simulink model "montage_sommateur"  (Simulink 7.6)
settings: Solver=ode15s  StartTime=0.0  StopTime=0.2  RelTol=1e-3
InitFcn:
  | Ad=10^5;
  | Vsat=15;
StopFcn:
  | close all, clc
  | load  ES_sommateur.mat
  | plot(x(1,:),x(2,:))
  | hold on
  | plot(x(1,:),x(3,:))
  | plot(x(1,:),x(4,:))
  | grid
  | title('Tensions d'entrée et de sortie - Montage sommateur')
  | xlabel('temps')
libraries: fl_lib x23, nesl_utility x4

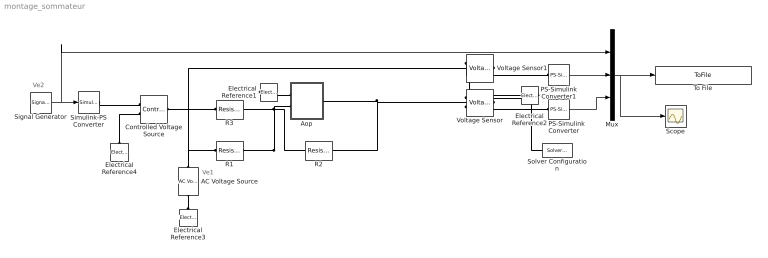
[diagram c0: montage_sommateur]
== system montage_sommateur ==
  note: Ve1
  note: Ve2
  AC Voltage Source : fl_lib/Electrical/Electrical Sources/AC Voltage Source  DialogController=NetworkEngine.DynNeDlgSource  SystemSampleTime=-1  amp=2 V  shift=0 rad  omega=10 Hz  i_Log=off  v_Log=off  LocalVarNames=|current|voltage|power  LocalVarDescs=|Current (A)|Voltage (V)|Power (W)  LocalVarLogging=[0 0 0]
  Aop : Subsystem
  Controlled Voltage Source : fl_lib/Electrical/Electrical Sources/Controlled Voltage Source  DialogController=NetworkEngine.DynNeDlgSource  SystemSampleTime=-1  i_Log=off  v_Log=off  LocalVarNames=|i|v  LocalVarDescs=|i|v  LocalVarLogging=[0 0]
  Electrical Reference{1..4} (4 alike) : fl_lib/Electrical/Electrical Elements/Electrical Reference  DialogController=NetworkEngine.DynNeDlgSource  SystemSampleTime=-1  i_Log=off  LocalVarNames=|i  LocalVarDescs=|i  LocalVarLogging=[]
  Mux : Mux  Inputs=3
  PS-Simulink Converter : nesl_utility/PS-Simulink Converter  DialogController=NetworkEngine.DynNeUtilDlgSource  SystemSampleTime=-1  PhysicalDomain=network_engine_domain  LeftPortType=input  RightPortType=output  SubClassName=ps_output  Unit=1  AffineConversion=off
  PS-Simulink Converter1 : nesl_utility/PS-Simulink Converter  DialogController=NetworkEngine.DynNeUtilDlgSource  SystemSampleTime=-1  PhysicalDomain=network_engine_domain  LeftPortType=input  RightPortType=output  SubClassName=ps_output  Unit=1  AffineConversion=off
  R1 : fl_lib/Electrical/Electrical Elements/Resistor  DialogController=NetworkEngine.DynNeDlgSource  SystemSampleTime=-1  R=10 kOhm  i_Log=off  v_Log=off  LocalVarNames=|current|voltage|power  LocalVarDescs=|Resistor current (A)|Voltage across resistor (V)|Power (W)  LocalVarLogging=[0 0 0]
  R2 : fl_lib/Electrical/Electrical Elements/Resistor  DialogController=NetworkEngine.DynNeDlgSource  SystemSampleTime=-1  R=10 kOhm  i_Log=off  v_Log=off  LocalVarNames=|current|voltage|power  LocalVarDescs=|Resistor current (A)|Voltage across resistor (V)|Power (W)  LocalVarLogging=[0 0 0]
  R3 : fl_lib/Electrical/Electrical Elements/Resistor  DialogController=NetworkEngine.DynNeDlgSource  SystemSampleTime=-1  R=10 kOhm  i_Log=off  v_Log=off  LocalVarNames=|current|voltage|power  LocalVarDescs=|Resistor current (A)|Voltage across resistor (V)|Power (W)  LocalVarLogging=[0 0 0]
  Scope : Scope
  Signal Generator : SignalGenerator  Frequency=20
  Simulink-PS Converter : nesl_utility/Simulink-PS Converter  DialogController=NetworkEngine.DynNeUtilDlgSource  SystemSampleTime=-1  PhysicalDomain=network_engine_domain  LeftPortType=input  RightPortType=output  SubClassName=ps_input  Unit=1  AffineConversion=off  InputFilterTimeConstant=.001  UdotUserProvided=0
  Solver Configuration : nesl_utility/Solver Configuration  DialogController=NetworkEngine.DynNeUtilDlgSource  SystemSampleTime=-1  PhysicalDomain=network_engine_domain  LeftPortType=input  RightPortType=generic  SubClassName=solver  Accelerate=off  Profile=off  ResidualTolerance=1e-9  MaxNonlinIter=12  MaxModeIter=2  DoFixedCost=off  UseLocalSampling=off  DoDC=off  LinearAlgebra=Sparse  LocalSolverSampleTime=.001  LocalSolverChoice=NE_BACKWARD_EULER_ADVANCER  UseLocalSolver=off
  To File : ToFile  Filename=ES_sommateur  MatrixName=x
  Voltage Sensor : fl_lib/Electrical/Electrical Sensors/Voltage Sensor  DialogController=NetworkEngine.DynNeDlgSource  SystemSampleTime=-1  i1_Log=off  v1_Log=off  LocalVarNames=|i1|v1  LocalVarDescs=|i1|v1  LocalVarLogging=[0 0]
  Voltage Sensor1 : fl_lib/Electrical/Electrical Sensors/Voltage Sensor  DialogController=NetworkEngine.DynNeDlgSource  SystemSampleTime=-1  i1_Log=off  v1_Log=off  LocalVarNames=|i1|v1  LocalVarDescs=|i1|v1  LocalVarLogging=[0 0]
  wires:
  Mux/1 -> To File/1, Scope/1
  Signal Generator/1 -> Simulink-PS Converter/1, Mux/1
  PS-Simulink Converter/1 -> Mux/3
  PS-Simulink Converter1/1 -> Mux/2
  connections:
  AC Voltage Source/RConn1 -- Electrical Reference3/LConn1
  Aop/RConn1 -- Voltage Sensor/LConn1 -- R2/RConn1
  Voltage Sensor/RConn1 -- PS-Simulink Converter/LConn1 -- Solver Configuration/RConn1
  Voltage Sensor/RConn2 -- Electrical Reference2/LConn1 -- Voltage Sensor1/RConn2
  R2/LConn1 -- R1/RConn1 -- Aop/LConn2 -- R3/RConn1
  Voltage Sensor1/RConn1 -- PS-Simulink Converter1/LConn1
  AC Voltage Source/LConn1 -- R1/LConn1 -- Voltage Sensor1/LConn1
  Electrical Reference1/LConn1 -- Aop/LConn1
  Controlled Voltage Source/LConn1 -- R3/LConn1
  Simulink-PS Converter/RConn1 -- Controlled Voltage Source/RConn1
  Electrical Reference4/LConn1 -- Controlled Voltage Source/RConn2

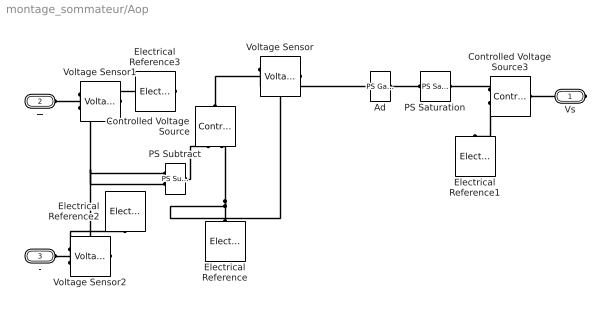
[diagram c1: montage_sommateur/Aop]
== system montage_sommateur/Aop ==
  Ad : fl_lib/Physical Signals/Functions/PS Gain  DialogController=NetworkEngine.DynNeDlgSource  SystemSampleTime=-1  gain=Ad  LocalVarLogging=[]
  Controlled Voltage Source : fl_lib/Electrical/Electrical Sources/Controlled Voltage Source  DialogController=NetworkEngine.DynNeDlgSource  SystemSampleTime=-1  i_Log=off  v_Log=off  LocalVarNames=|i|v  LocalVarDescs=|i|v  LocalVarLogging=[0 0]
  Controlled Voltage Source3 : fl_lib/Electrical/Electrical Sources/Controlled Voltage Source  DialogController=NetworkEngine.DynNeDlgSource  SystemSampleTime=-1  i_Log=off  v_Log=off  LocalVarNames=|i|v  LocalVarDescs=|i|v  LocalVarLogging=[0 0]
  Electrical Reference{,1..3} (4 alike) : fl_lib/Electrical/Electrical Elements/Electrical Reference  DialogController=NetworkEngine.DynNeDlgSource  SystemSampleTime=-1  i_Log=off  LocalVarNames=|i  LocalVarDescs=|i  LocalVarLogging=0
  PS Saturation : fl_lib/Physical Signals/Nonlinear Operators/PS Saturation  DialogController=NetworkEngine.DynNeDlgSource  SystemSampleTime=-1  upper_limit=Vsat  lower_limit=-Vsat  LocalVarLogging=[]
  PS Subtract : fl_lib/Physical Signals/Functions/PS Subtract  DialogController=NetworkEngine.DynNeDlgSource  SystemSampleTime=-1  LocalVarLogging=[]
  Voltage Sensor : fl_lib/Electrical/Electrical Sensors/Voltage Sensor  DialogController=NetworkEngine.DynNeDlgSource  SystemSampleTime=-1  i1_Log=off  v1_Log=off  LocalVarNames=|i1|v1  LocalVarDescs=|i1|v1  LocalVarLogging=[0 0]
  Voltage Sensor1 : fl_lib/Electrical/Electrical Sensors/Voltage Sensor  DialogController=NetworkEngine.DynNeDlgSource  SystemSampleTime=-1  i1_Log=off  v1_Log=off  LocalVarNames=|i1|v1  LocalVarDescs=|i1|v1  LocalVarLogging=[0 0]
  Voltage Sensor2 : fl_lib/Electrical/Electrical Sensors/Voltage Sensor  DialogController=NetworkEngine.DynNeDlgSource  SystemSampleTime=-1  i1_Log=off  v1_Log=off  LocalVarNames=|i1|v1  LocalVarDescs=|i1|v1  LocalVarLogging=[0 0]
  Vs : PMIOPort  Port=1  Side=Right
  + : PMIOPort  Port=2  Side=Left
  - : PMIOPort  Port=3  Side=Left
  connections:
  Voltage Sensor/RConn1 -- Ad/LConn1
  PS Saturation/LConn1 -- Ad/RConn1
  Controlled Voltage Source/LConn1 -- Voltage Sensor/LConn1
  PS Subtract/RConn1 -- Controlled Voltage Source/RConn1
  Electrical Reference/LConn1 -- Controlled Voltage Source/RConn2 -- Voltage Sensor/RConn2
  Controlled Voltage Source3/RConn1 -- PS Saturation/RConn1
  Controlled Voltage Source3/RConn2 -- Electrical Reference1/LConn1
  Vs/RConn1 -- Controlled Voltage Source3/LConn1
  +/RConn1 -- Voltage Sensor1/LConn1
  -/RConn1 -- Voltage Sensor2/LConn1
  Voltage Sensor2/RConn1 -- PS Subtract/LConn2
  Voltage Sensor1/RConn1 -- PS Subtract/LConn1
  Voltage Sensor1/RConn2 -- Electrical Reference3/LConn1
  Voltage Sensor2/RConn2 -- Electrical Reference2/LConn1
